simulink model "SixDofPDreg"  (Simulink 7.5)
settings: Solver=ode45  StartTime=0.0  StopTime=5  RelTol=1e-6

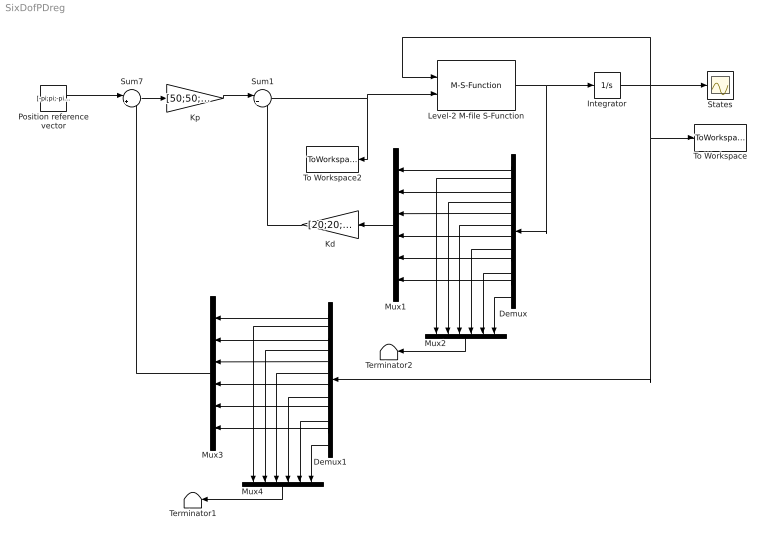
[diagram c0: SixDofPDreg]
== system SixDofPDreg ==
  Demux : Demux  Outputs=12
  Demux1 : Demux  Outputs=12
  Integrator : Integrator  InitialCondition=[0; 0; pi/2; 0; -pi/2; 0; 0; 0; 0; 0; 0; 0;]  AbsoluteTolerance=1e-10
  Kd : Gain  Gain=[20;20;20;20;20;22]  ParameterDataType=fixdt(1, 16)  ParameterScaling=2^0  OutDataType=fixdt(1, 16)  OutScaling=2^0
  Kp : Gain  Gain=[50;50;50;50;50;60]  ParameterDataType=fixdt(1, 16)  ParameterScaling=2^0  OutDataType=fixdt(1, 16)  OutScaling=2^0
  Level-2 M-file S-Function : M-S-Function  FunctionName=irb140
  Mux{1..4} (4 alike) : Mux  Inputs=6
  Position reference vector : Constant  Value=[-pi;pi;-pi;-pi;-pi/2;pi]  OutDataType=fixdt(1, 16)  OutScaling=2^0
  States : Scope
  Sum1 : Sum  Inputs=|+-  OutDataType=fixdt(1, 16)  OutScaling=2^0
  Sum7 : Sum  Inputs=|+-  OutDataType=fixdt(1, 16)  OutScaling=2^0
  Terminator1 : Terminator
  Terminator2 : Terminator
  To Workspace : ToWorkspace  VariableName=states  SampleTime=-1  SaveFormat=Structure With Time
  To Workspace2 : ToWorkspace  VariableName=tau  SampleTime=-1  SaveFormat=Structure With Time
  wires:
  Integrator/1 -> Level-2 M-file S-Function/1, States/1, To Workspace/1, Demux1/1
  Level-2 M-file S-Function/1 -> Integrator/1, Demux/1
  Demux/1 -> Mux1/1
  Demux/3 -> Mux1/2
  Demux/5 -> Mux1/3
  Demux/7 -> Mux1/4
  Demux/9 -> Mux1/5
  Demux/11 -> Mux1/6
  Demux/12 -> Mux2/6
  Demux/10 -> Mux2/5
  Demux/8 -> Mux2/4
  Demux/6 -> Mux2/3
  Demux/4 -> Mux2/2
  Demux/2 -> Mux2/1
  Mux2/1 -> Terminator2/1
  Mux1/1 -> Kd/1
  Kd/1 -> Sum1/2
  Demux1/1 -> Mux3/1
  Demux1/3 -> Mux3/2
  Demux1/5 -> Mux3/3
  Demux1/7 -> Mux3/4
  Demux1/9 -> Mux3/5
  Demux1/11 -> Mux3/6
  Demux1/12 -> Mux4/6
  Demux1/10 -> Mux4/5
  Demux1/8 -> Mux4/4
  Demux1/6 -> Mux4/3
  Demux1/4 -> Mux4/2
  Demux1/2 -> Mux4/1
  Mux4/1 -> Terminator1/1
  Mux3/1 -> Sum7/2
  Sum7/1 -> Kp/1
  Kp/1 -> Sum1/1
  Position reference vector/1 -> Sum7/1
  Sum1/1 -> Level-2 M-file S-Function/2, To Workspace2/1
